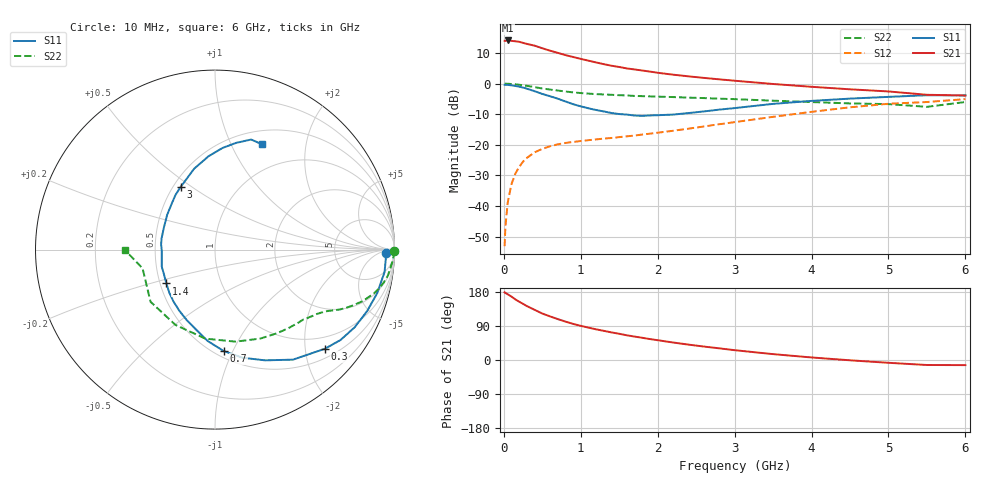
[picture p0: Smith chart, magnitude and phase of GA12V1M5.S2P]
! Infineon Technologies  Discrete & RF Semiconductors
! BF775
! Si NPN RF Bipolar Junction Transistor in SOT23
! VCE = 12 V  IC = 1.5 mA
! Common Emitter S-Parameters:  May  1996
# GHz  S  MA  R  50
!  f  S11  S21  S12  S22
! GHz  MAG  ANG  MAG  ANG  MAG  ANG  MAG  ANG
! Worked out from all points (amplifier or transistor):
!   36 points, 10 MHz to 6 GHz, reference 50 ohm
!   highest |S21| = 14.1 dB at 50 MHz (marker M1)
!   |S21| within 3 dB of that: start of sweep to 556.9 MHz
!   unconditionally stable (mu >= 1): 1.334 GHz to 3.208 GHz
!   at 250 MHz: K = 0.24, MSG = 19.4 dB, |S12| = -25.5 dB
!   at 1.4 GHz: K = 1.03, MAG = 10.7 dB, |S12| = -17.8 dB
!   at 6 GHz: K = 0.94, MSG = 0.6 dB, |S12| = -5.1 dB
!   S11 on the Smith chart (normalised r, x): 10 MHz: 35, -17; 300 MHz: 0.70, -2.42; 700 MHz: 0.55, -0.92; 1.4 GHz: 0.54, -0.23; 3 GHz: 0.55, +0.45; 6 GHz: 0.66, +1.32
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0.01  0.9552 -1.3  4.994 178.8  0.0022 84.8  0.9999 -0.6
0.02  0.9531 -2.8  4.976 177.1  0.0045 89.5  0.9952 -1.1
0.05  0.953 -7.5  5.069 173.4  0.0113 84.0  0.9947 -2.9
0.1  0.9358 -15.0  4.992 167.2  0.0229 80.4  0.9833 -5.8
0.15  0.914 -22.1  4.912 159.9  0.0338 76.1  0.9737 -8.6
0.2  0.8903 -29.1  4.823 153.8  0.0435 73.1  0.9572 -11.1
0.3  0.8244 -42.1  4.451 142.2  0.0611 65.8  0.9184 -15.4
0.4  0.7513 -54.7  4.165 132.4  0.0752 60.0  0.8747 -19.0
0.5  0.677 -65.7  3.779 122.6  0.0857 55.3  0.8313 -21.9
0.6  0.6214 -75.8  3.451 115.1  0.0944 51.7  0.7986 -24.0
0.7  0.5672 -85.1  3.179 108.0  0.1016 49.3  0.7705 -25.7
0.9  0.4605 -102.8  2.721 95.3  0.1113 46.0  0.7182 -28.4
1.1  0.3944 -120.3  2.369 85.5  0.1188 44.7  0.6857 -30.9
1.4  0.3301 -145.1  1.957 72.8  0.1291 44.8  0.6554 -34.5
1.7  0.3002 -171.4  1.703 61.8  0.1414 47.1  0.6282 -38.3
2.2  0.3113 155.6  1.398 46.2  0.1693 50.2  0.6019 -46.0
3  0.3975 118.9  1.114 25.9  0.2343 51.7  0.5566 -62.9
3.5  0.4658 104.4  0.985 15.5  0.286 49.2  0.5253 -77.5
4.5  0.5683 85.7  0.806 -0.8  0.4095 38.8  0.474 -117.7
5  0.6061 78.8  0.744 -7.4  0.4679 30.9  0.462 -141.0
5.5  0.6456 71.8  0.656 -13.2  0.4996 21.4  0.4168 -165.5
6  0.6423 66.1  0.638 -13.5  0.5574 16.5  0.4998 -179.5
